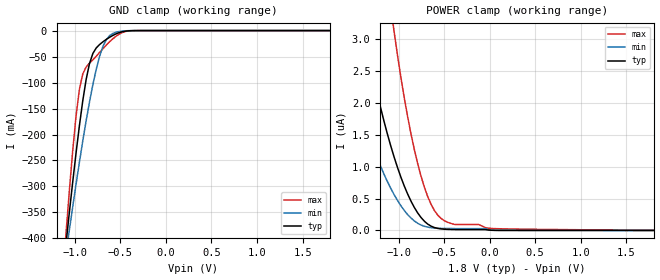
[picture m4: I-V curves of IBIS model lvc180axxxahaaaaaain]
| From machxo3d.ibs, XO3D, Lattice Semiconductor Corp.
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|   Model lvc180axxxahaaaaaain
[Model] lvc180axxxahaaaaaain
Model_type Input
Polarity   Non-Inverting
Enable   Active-High
Vinl =  0.630V
Vinh =  1.170V
C_comp   4.200pF   3.800pF   7.500pF
[Temperature Range]   25.000   0.105k   -40.000
[Voltage Range]   1.800V   1.710V   1.890V
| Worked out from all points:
|   GND clamp passes 1 mA (typ) near -0.44 V on its own axis
[GND_clamp]
|Voltage   I(typ)   I(min)   I(max)
-1.8V     -1.677A    -1.372A    -2.207A
-1.097V   -411.6mA   -430.5mA   -392.9mA
-1.06V    -351mA     -384.7mA   -309.8mA
-986mV    -235.9mA   -295.9mA   -164.7mA
-949mV    -183mA     -253.4mA   -113mA
-912mV    -135mA     -212.5mA   -83.33mA
-838mV    -63.16mA   -137.2mA   -62.66mA
-801mV    -43.93mA   -103.8mA   -56.25mA
-690mV    -21.49mA   -30.06mA   -34.72mA
-579mV    -9.043mA   -5.343mA   -15.31mA
-357mV    -110.3uA   -52.32uA   -166.6uA
1.8V      0A         0A         0A
[POWER_clamp]
|Voltage   I(typ)   I(min)   I(max)
-1.8V     6.918uA    4.075uA    15.53uA
-1.641V   5.335uA    3.081uA    12.17uA
-1.382V   3.16uA     1.741uA    7.507uA
-1.197V   1.931uA    1.01uA     4.843uA
-1.049V   1.156uA    564.3nA    3.128uA
-901mV    576.3nA    251.8nA    1.796uA
-790mV    276.2nA    113.3nA    1.051uA
-679mV    99.59nA    51.82nA    530.4nA
-605mV    45.38nA    37.94nA    310.9nA
-420mV    15.41nA    30.13nA    108.3nA
61mV      1.594nA    2.49nA     28.82nA
1.8V      0A         0A         4.229nA
